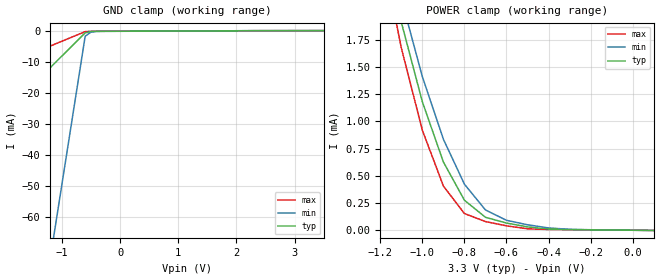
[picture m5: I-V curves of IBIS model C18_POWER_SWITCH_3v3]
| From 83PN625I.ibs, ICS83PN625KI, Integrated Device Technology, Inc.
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[Model] C18_POWER_SWITCH_3v3
Model_type   Input
Polarity   Non-Inverting
Vinl = 0.8V
Vinh = 2.0V
|   typ   min   max
C_comp   2pF   1.5pF   2.5pF
|   typ   min   max
[Voltage range]   3.3V   3.135V   3.465V
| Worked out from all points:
|   GND clamp passes 1 mA (typ) near -0.61 V on its own axis
|   POWER clamp passes 1 mA (typ) near -0.97 V on its own axis
[GND_clamp]
|Voltage   I (typ)   I (min)   I (max)
-3.3V     -51.02mA   -323.8mA   -21.16mA
-1.2V     -11.9mA    -73.33mA   -4.953mA
-1.1V     -10.04mA   -61.41mA   -4.181mA
-600mV    -721.5uA   -1.785mA   -323.1uA
-500mV    -290.1uA   -488.1uA   -210.5uA
-300mV    -216.8uA   -234.2uA   -193uA
3.5V      4.001uA    14.8uA     595.6nA
[Power_clamp]
|Voltage   I (typ)   I (min)   I (max)
-3.3V     42.96mA    38.61mA    50.07mA
-1.2V     2.802mA    2.968mA    2.645mA
-1.1V     1.91mA     2.125mA    1.674mA
-1V       1.179mA    1.41mA     918.2uA
-900mV    626.5uA    835.5uA    405.4uA
-800mV    275.5uA    422.7uA    153.3uA
-700mV    118.8uA    186.1uA    79.69uA
-600mV    65.78uA    91.21uA    40.34uA
-500mV    30.67uA    50.18uA    13.23uA
-400mV    10.84uA    21.25uA    6.941uA
-300mV    6.12uA     8.219uA    5.107uA
100mV     -1.999uA   -2.241uA   -1.702uA
